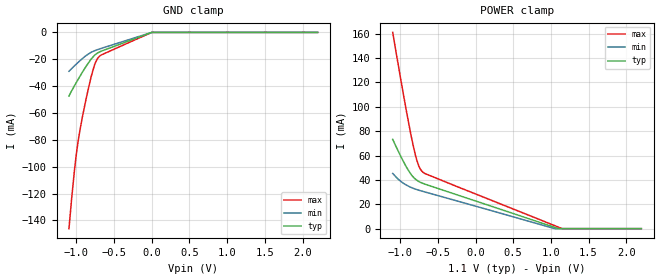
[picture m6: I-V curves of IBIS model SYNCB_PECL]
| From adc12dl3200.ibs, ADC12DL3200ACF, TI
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|   Model SYNCB_PECL
[Model]   SYNCB_PECL
Model_type   Input
Vinl = .57
Vinh = 1.33
|   (nom PVT)   (fast PVT)   (slow PVT)
|   typ   min   max
C_comp   0.804p   0.760p   0.851p
[Voltage Range]   1.1   1.05   1.15
[Temperature Range]   27   125   -40
[Power Clamp Reference]   1.1   1.05   1.15
[GND Clamp Reference]   0   0   0
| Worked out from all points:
|   GND clamp passes 1 mA (typ) near -0.05 V on its own axis
[GND Clamp]
|   Voltage   I(typ)   I(min)   I(max)
-1.1V     -47.36mA   -28.94mA   -146.1mA
-1.064V   -43.44mA   -26.91mA   -123.4mA
-1.027V   -39.78mA   -24.92mA   -102.9mA
-1.001V   -37.18mA   -23.5mA    -90.19mA
-968mV    -34mA      -21.78mA   -77.28mA
-888.8mV  -26.68mA   -17.97mA   -53.87mA
-803mV    -19.72mA   -14.77mA   -32.52mA
-753.5mV  -16.73mA   -13.51mA   -23.17mA
-723.8mV  -15.47mA   -12.89mA   -19.64mA
-697.4mV  -14.65mA   -12.38mA   -17.86mA
-1.1mV    -22.9uA    -19.5uA    -27.67uA
2.2V      0A         0A         0A
[POWER Clamp]
|   Voltage   I(typ)   I(min)   I(max)
-1.1V     73.25mA    45.31mA    161mA
-997.7mV  59.95mA    39.02mA    124.1mA
-925.1mV  51.31mA    35.98mA    98.86mA
-872.3mV  45.92mA    34.29mA    81.5mA
-836mV    42.96mA    33.31mA    70.44mA
-796.4mV  40.55mA    32.41mA    59.87mA
-753.5mV  38.72mA    31.56mA    51.44mA
-737mV    38.17mA    31.26mA    49.29mA
-697.4mV  37.1mA     30.55mA    46.24mA
1.048V    1.071mA    30.02uA    2.521mA
1.147V    0A         0A         66.58uA
2.2V      0A         0A         0A
